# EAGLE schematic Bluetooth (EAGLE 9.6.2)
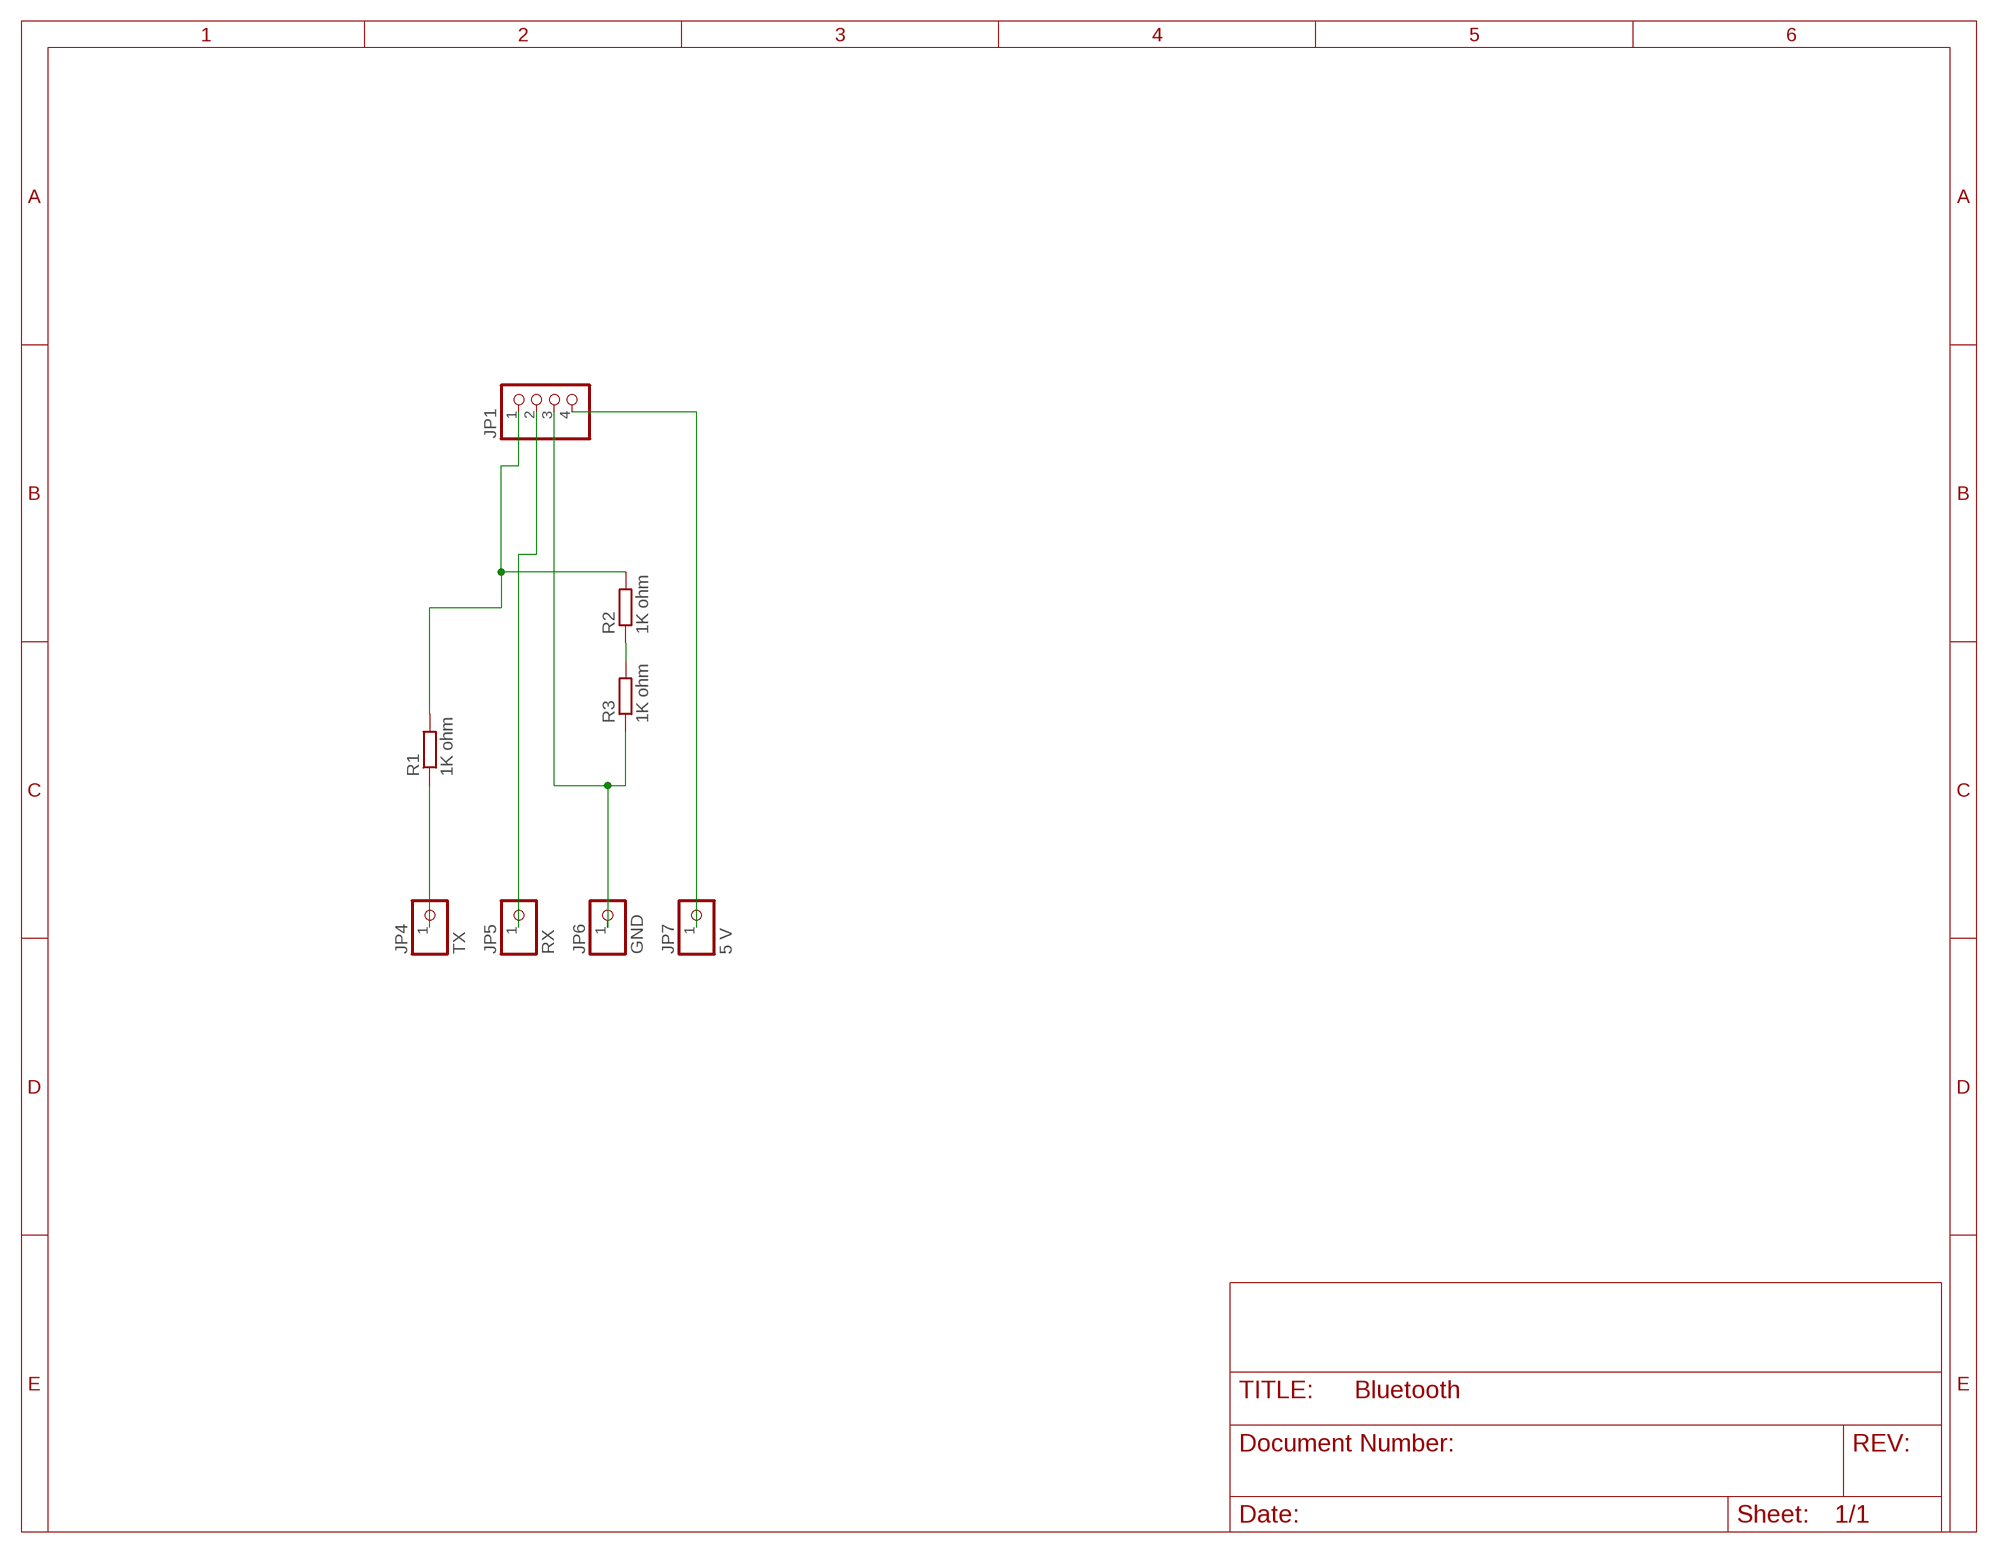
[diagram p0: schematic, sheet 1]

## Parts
JP1  PINHD-1X4  [1X04]
JP4  TX  PINHD-1X1  [1X01]
JP5  RX  PINHD-1X1  [1X01]
JP6  GND  PINHD-1X1  [1X01]
JP7  5 V  PINHD-1X1  [1X01]
R1  1K ohm  R-EU_VMTA55  [VMTA55]
R2  1K ohm  R-EU_VMTA55  [VMTA55]
R3  1K ohm  R-EU_VMTA55  [VMTA55]

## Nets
N$1: JP1.4 JP7.1
N$2: JP4.1 R1.1
N$3: JP1.2 JP5.1
N$4: JP1.1 R1.2 R2.2
N$5: JP1.3 JP6.1 R3.1
N$6: R2.1 R3.2

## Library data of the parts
JP1 = pinhead:PINHD-1X4: PIN HEADER
JP4-JP7 = pinhead:PINHD-1X1: PIN HEADER
R1-R3 = rcl:R-EU_: RESISTOR, European symbol; SPICEPREFIX: R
